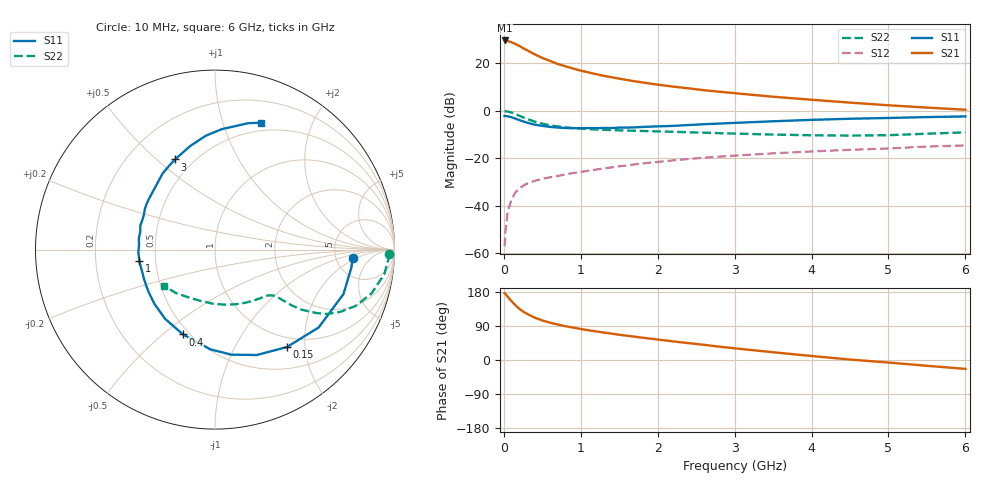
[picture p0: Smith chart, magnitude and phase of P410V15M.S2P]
! SIEMENS Small Signal Semiconductors
! BFP182
! Si NPN RF Bipolar Junction Transistor in SOT143
! VCE = 10 V  IC = 15 mA
! Common Emitter S-Parameters:  March  1996
# GHz  S  MA  R  50
!  f  S11  S21  S12  S22
! GHz  MAG  ANG  MAG  ANG  MAG  ANG  MAG  ANG
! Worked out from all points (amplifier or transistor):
!   36 points, 10 MHz to 6 GHz, reference 50 ohm
!   highest |S21| = 29.5 dB at 10 MHz (marker M1)
!   |S21| within 3 dB of that: start of sweep to 237.8 MHz
!   unconditionally stable (mu >= 1): 1.111 GHz to 5.76 GHz
!   at 250 MHz: K = 0.38, MSG = 29.0 dB, |S12| = -31.7 dB
!   at 1.4 GHz: K = 1.08, MAG = 17.2 dB, |S12| = -23.9 dB
!   at 6 GHz: K = 0.98, MSG = 7.5 dB, |S12| = -14.7 dB
!   S11 on the Smith chart (normalised r, x): 10 MHz: 7.20, -1.74; 150 MHz: 0.83, -1.66; 400 MHz: 0.46, -0.59; 1 GHz: 0.40, -0.06; 3 GHz: 0.40, +0.58; 6 GHz: 0.41, +1.34
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0.01  0.7682 -3.7  29.82 176.3  0.0014 73.5  0.9673 -1.4
0.02  0.7663 -7.5  29.81 174.5  0.0028 82.9  0.9677 -3.2
0.05  0.7574 -19.1  29.09 166.9  0.0075 82.6  0.9534 -8.2
0.1  0.7224 -36.9  27.29 155.2  0.0134 71.3  0.9053 -15.7
0.15  0.6748 -53.6  25.18 144.5  0.0189 65.0  0.8433 -21.9
0.2  0.6316 -68.4  22.89 135.5  0.0229 59.3  0.7799 -26.4
0.25  0.5925 -81.1  20.56 127.9  0.026 56.1  0.7193 -29.9
0.3  0.5566 -92.6  18.63 122.0  0.029 53.3  0.6654 -32.1
0.4  0.5051 -110.7  15.27 111.9  0.0331 50.2  0.5855 -34.8
0.5  0.4757 -125.6  12.77 104.4  0.0365 48.3  0.5295 -36.0
0.6  0.4532 -138.0  11.06 98.5  0.0394 48.0  0.4901 -36.5
0.7  0.4388 -147.7  9.564 93.6  0.042 47.9  0.4627 -36.9
0.8  0.4293 -156.2  8.538 89.2  0.0452 48.1  0.4426 -37.2
1  0.4261 -171.5  6.908 81.8  0.051 48.2  0.4162 -38.1
1.1  0.4275 -177.9  6.342 78.4  0.0543 48.5  0.4068 -38.8
1.5  0.4369 162.4  4.683 66.6  0.067 48.0  0.383 -42.5
2.2  0.4755 136.2  3.188 49.1  0.0893 44.4  0.3574 -52.7
3  0.5496 113.9  2.318 30.9  0.1126 38.3  0.3276 -68.1
3.5  0.5938 103.4  1.952 20.4  0.1255 33.9  0.3123 -79.5
4.5  0.6716 86.9  1.467 1.2  0.149 25.6  0.297 -105.5
5.5  0.7281 75.3  1.154 -15.3  0.1743 18.3  0.3251 -131.6
6  0.752 70.1  1.04 -23.4  0.1846 13.6  0.3477 -144.2
